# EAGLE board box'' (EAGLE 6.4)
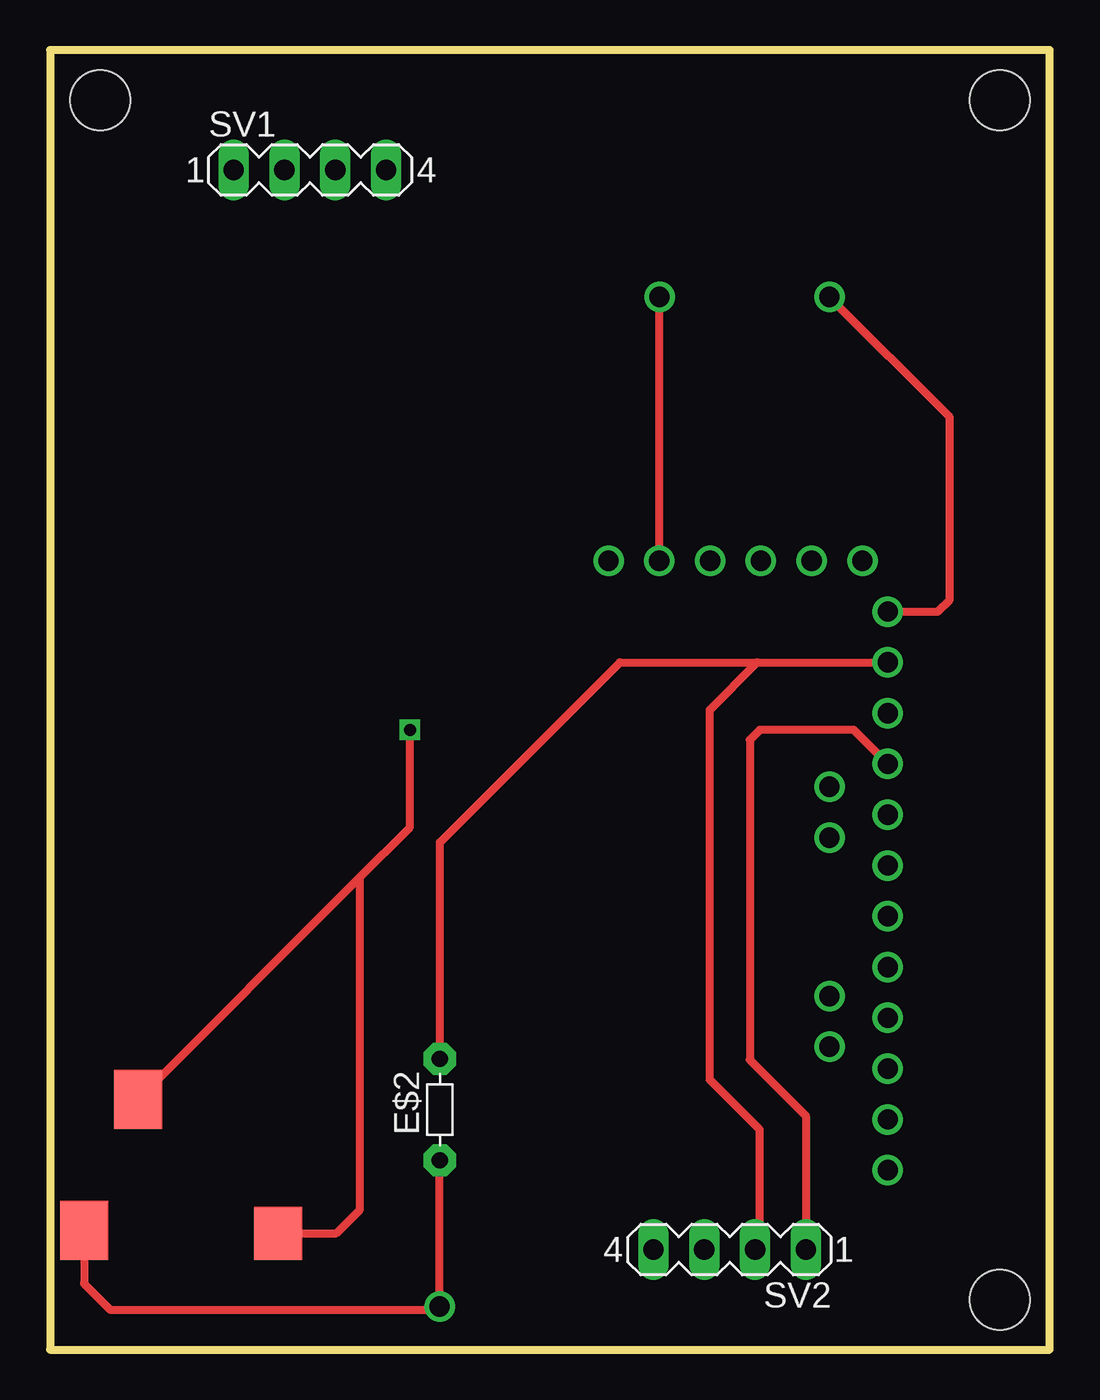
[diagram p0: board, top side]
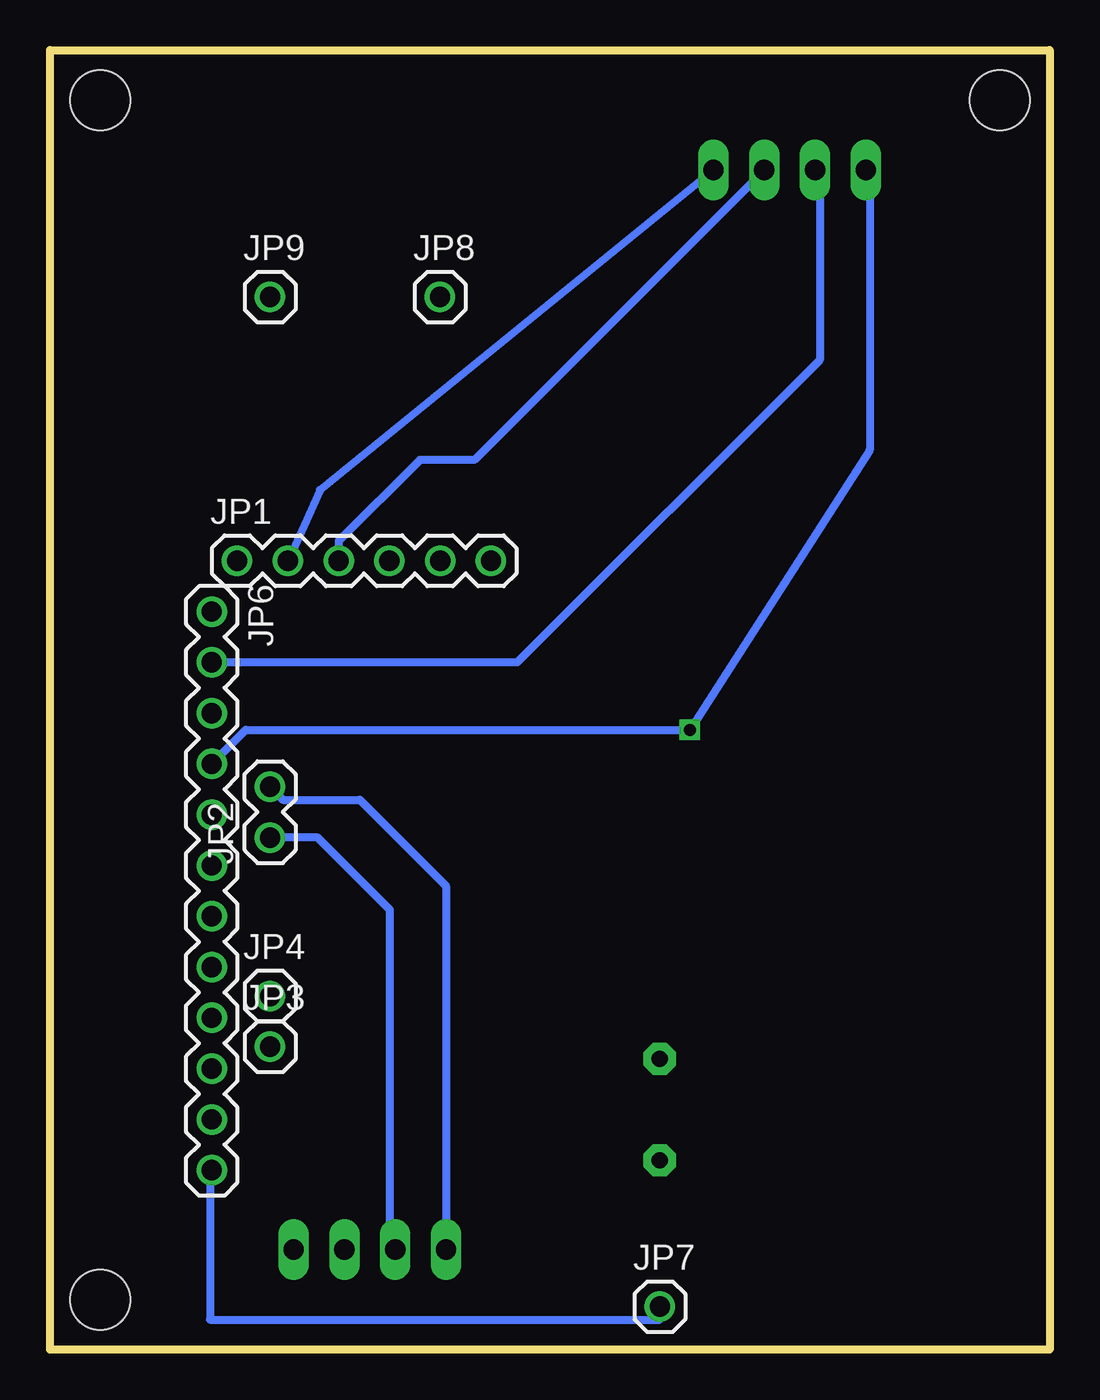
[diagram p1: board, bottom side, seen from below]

Size 50 x 65 mm. Coordinates in mm from the lower left corner, seen from the top.
Outline: 0,0 50,0 50,65 0,65 0,0
Copper layers (1*16): Top 0.035mm / dielectric 1.5mm / Bottom 0.035mm
Design rules "default": minimum track width 10mil, minimum drill 24mil, track to track 8mil, track to pad 8mil, pad to pad 8mil, via to via 8mil, smd to smd 8mil, copper to edge 40mil, drill to drill 8mil, minimum pad ring 10mil, minimum via ring 8mil, stop-mask expansion 4mil, vias tented up to drill 0mil, thermal gap 10mil
Net classes: 0 default: width 0.203 mm; 1 vcc: width 0.254 mm
Holes 3 mm at 47.5,2.5 2.5,62.5 47.5,62.5

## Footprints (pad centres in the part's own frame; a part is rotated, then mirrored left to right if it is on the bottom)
SMDAUDIO = smd 2.4 x 2.95: P$1 1.7,1.475; P$2 4.4,8.025 | smd 2.4 x 2.65: P$3 11.4,1.325
R-5 = drill 0.813 pad 1.6 octagon: 1 -2.54,0; 2 2.54,0
1X06 = drill 1.016: 1 0,0; 2 2.54,0; 3 5.08,0; 4 7.62,0; 5 10.16,0; 6 12.7,0
1X02 = drill 1.016: 1 0,0; 2 2.54,0
1X01 = drill 1.016: 1 0,0
1X12 = drill 1.016: 1 0,0; 2 2.54,0; 3 5.08,0; 4 7.62,0; 5 10.16,0; 6 12.7,0; 7 15.24,0; 8 17.78,0; 9 20.32,0; 10 22.86,0; 11 25.4,0; 12 27.94,0
MA04-1 = drill 1.016 long: 1 -3.81,0; 2 -1.27,0; 3 1.27,0; 4 3.81,0

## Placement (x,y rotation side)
E$1  [SMDAUDIO]  0,4.5 0 top
E$2  [R-5]  19.5,12 90 top
JP1  FTDI Basic  [1X06]  40.64,39.45 0 bottom
JP2  [1X02]  38.99,25.61 90 bottom
JP3  [1X01]  38.99,15.14 0 bottom
JP4  [1X01]  38.99,17.68 0 bottom
JP6  [1X12]  41.91,36.91 270 bottom
JP7  [1X01]  19.49,2.14 0 bottom
JP8  [1X01]  30.49,52.64 0 bottom
JP9  [1X01]  38.99,52.64 0 bottom
SV1  [MA04-1]  13,59 0 top
SV2  [MA04-1]  34,5 180 top

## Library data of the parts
E$1 = audiojack
E$2 = discrete
JP1-JP4 JP6-JP9 = SparkFun
SV1 SV2 = con-lstb; OC_FARNELL: unknown; OC_NEWARK: unknown

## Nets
S$1: JP1.2 SV1.4
S$2: JP1.3 SV1.3
S$3: JP2.2 SV2.4
S$4: JP2.1 SV2.3
S$5: E$2.2 JP6.2 SV1.2 SV2.2
S$6: E$1.P$2 E$1.P$3 JP6.4 SV1.1 SV2.1
S$7: JP1.5 JP8.1
S$8: JP6.1 JP9.1
S$10: E$1.P$1 E$2.1 JP6.12 JP7.1

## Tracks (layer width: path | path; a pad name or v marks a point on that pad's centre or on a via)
S$1
  Bottom 0.406: SV1.4 36.5,43 JP1.2
S$2
  Bottom 0.406: SV1.3 28.77,44.5 31.5,44.5 35.56,40.44 JP1.3
S$3
  Bottom 0.406: JP2.2 38.34,27.5 34.5,27.5 30.19,23.19 SV2.4
S$4
  Bottom 0.406: SV2.3 33,5.27 33,22 36.61,25.61 JP2.1
S$5
  Top 0.406: SV2.2 35.5,5.23 35.5,11 33,13.5 33,32 35.37,34.37 JP6.2 28.5,34.37 19.5,25.37 E$2.2
  Bottom 0.406: SV1.2 11.5,58.77 11.5,49.5 26.63,34.37 JP6.2
S$6  (via drill 0.6)
  Top 0.406: JP6.4 40.2,31 35.5,31 35,30.5 35,14.5 37.81,11.69 SV2.1 | E$1.P$2 15.44,23.56 | 15.44,23.56 18,26.12 v18,31 | E$1.P$3 14.32,5.82 15.5,7 15.5,23.5 15.44,23.56
  Bottom 0.406: SV1.1 9,58.81 9,45 v18,31 40.2,31 JP6.4
S$7
  Top 0.406: JP1.5 JP8.1
S$8
  Top 0.406: JP6.1 44.41,36.91 45,37.5 45,46.63 JP9.1
S$10
  Top 0.406: E$1.P$1 1.7,3.3 3,2 19.35,2 JP7.1 E$2.1
  Bottom 0.406: JP6.12 42,8.97 42,1.5 19.49,1.5 JP7.1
